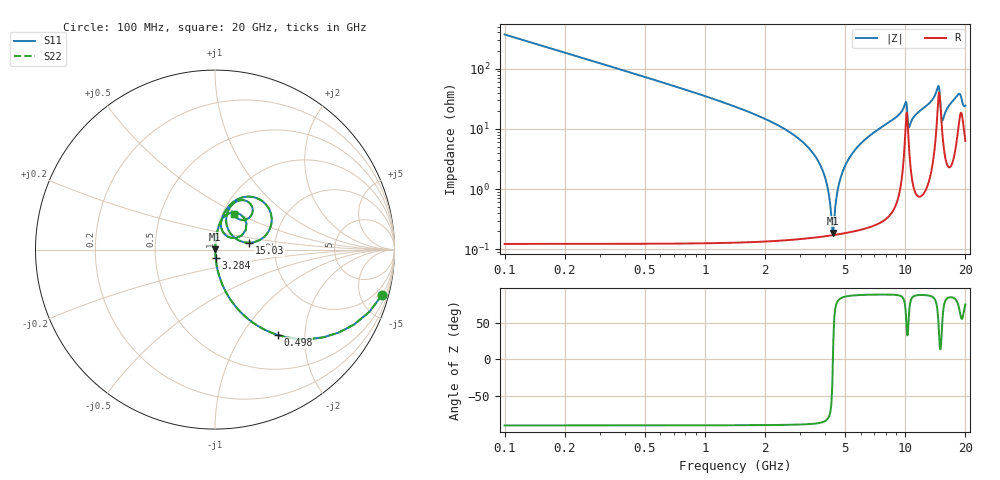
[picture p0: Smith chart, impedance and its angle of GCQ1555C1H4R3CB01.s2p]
!Murata Part Number: GCQ1555C1H4R3CB01
!These Parameters are Measured in Series Mode Connection
!Data Generated on Mar 13, 2026
!  o--ll--o
!Port1  Port2
!  o------o
!Operation Temp=25[degC], DC Bias Voltage=0[V]
!Freq. Start=100[MHz] Stop=20[GHz] 401[Steps]
# Hz S RI R 50
!Freq.(Hz) S11(Real) S11(Imag) S21(Real) S21(Imag) S12(Real) S12(Imag) S22(Real) S22(Imag)
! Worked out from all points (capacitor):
!   401 points, 100 MHz to 20 GHz, reference 50 ohm
!   read as one part in series: C = 4.3 pF near 199.5 MHz
!   lowest |Z| = 187 mohm at 4.378 GHz (marker M1)
!   series resonance near 4.36 GHz, so ESL is about 310 pH
!   S11 on the Smith chart (normalised r, x): 100 MHz: 1.00, -7.40; 498 MHz: 1.00, -1.47; 3.284 GHz: 1.00, -0.10; 15.03 GHz: 1.47, +0.12; 20 GHz: 1.13, +0.47
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1e8  0.9318 -0.2519  0.0682 0.2519  0.0682 0.2519  0.9318 -0.2519
4.98e8  0.3501 -0.4762  0.6499 0.4762  0.6499 0.4762  0.3501 -0.4762
1.24425e9  0.0706 -0.2539  0.9294 0.2539  0.9294 0.2539  0.0706 -0.2539
3.284e9  0.00392 -0.0489  0.9961 0.0489  0.9961 0.0489  0.00392 -0.0489
3.43325e9  0.00324 -0.0411  0.9968 0.0411  0.9968 0.0411  0.00324 -0.0411
3.9805e9  0.00189 -0.0156  0.9981 0.0156  0.9981 0.0156  0.00189 -0.0156
4.12975e9  0.00176 -0.0093  0.9982 0.0093  0.9982 0.0093  0.00176 -0.0093
4.279e9  0.00171 -0.00321  0.9983 0.00321  0.9983 0.00321  0.00171 -0.00321
4.3785e9  0.00172 0.000731  0.9983 -0.000731  0.9983 -0.000731  0.00172 0.000731
4.677e9  0.00193 0.0121  0.9981 -0.0121  0.9981 -0.0121  0.00193 0.0121
5.02525e9  0.00246 0.0246  0.9975 -0.0246  0.9975 -0.0246  0.00246 0.0246
6.7665e9  0.00878 0.0797  0.9912 -0.0797  0.9912 -0.0797  0.00878 0.0797
1.005e10  0.1395 0.1977  0.8605 -0.1977  0.8605 -0.1977  0.1395 0.1977
1.0448e10  0.0568 0.0828  0.9432 -0.0828  0.9432 -0.0828  0.0568 0.0828
1.1244e10  0.0358 0.1618  0.9642 -0.1618  0.9642 -0.1618  0.0358 0.1618
1.338325e10  0.0854 0.2508  0.9146 -0.2508  0.9146 -0.2508  0.0854 0.2508
1.4627e10  0.2997 0.2299  0.7003 -0.2299  0.7003 -0.2299  0.2997 0.2299
1.5025e10  0.191 0.038  0.809 -0.038  0.809 -0.038  0.191 0.038
1.53235e10  0.0897 0.0858  0.9103 -0.0858  0.9103 -0.0858  0.0897 0.0858
1.67165e10  0.0787 0.2275  0.9213 -0.2275  0.9213 -0.2275  0.0787 0.2275
1.85075e10  0.1881 0.2633  0.8119 -0.2633  0.8119 -0.2633  0.1881 0.2633
2e10  0.1032 0.1984  0.8968 -0.1984  0.8968 -0.1984  0.1032 0.1984
